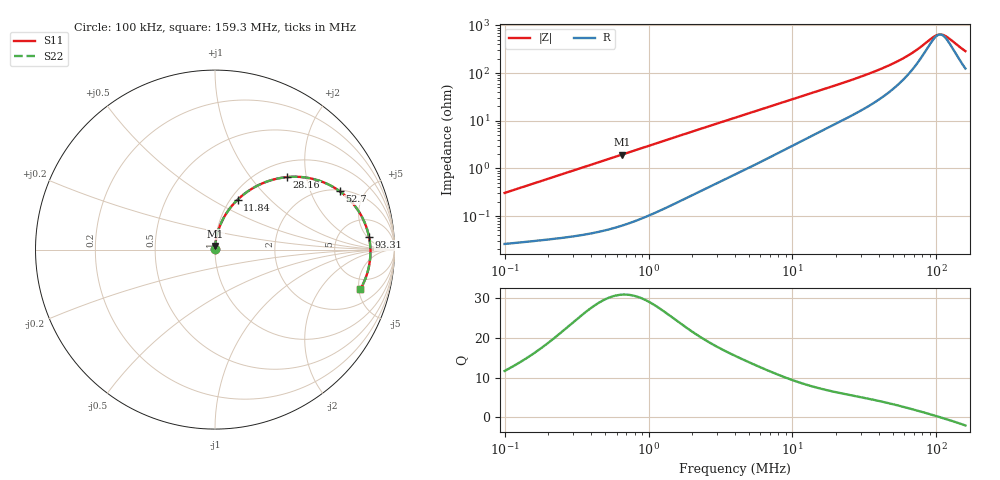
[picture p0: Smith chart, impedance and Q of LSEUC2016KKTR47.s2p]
! LSEUC2016KKTR47  S-PARAMETER MODEL  ( General Type )
! Model Generated by TAIYO YUDEN Corporation (http://www.ty-top.com)
! Version 1.0
! TAIYO YUDEN Control No. 220210
! Copyright(c) 2022 TAIYO YUDEN CO.,LTD. All Rights Reserved.
! Product Description (link to TY-COMPAS)
! https://ds.yuden.co.jp/TYCOMPAS/or/detail?pn=LSEUC2016KKTR47M&u=M
! Products Name : Inductors
! Characteristics :
!  Inductance : 0.47 uH , SRF(min) : -Hz , DC Resistance(max) : 0.026 Ohm
!  Rated Current : Saturation :6300 mA , Temp Rise : 4700 mA (40 degC)
!  Case Size : 2.0 x 1.6 / 0.079 x 0.063 [mm/inch] , Thickness : 1 / 0.039 [mm/inch]
!  (Conditions: Temperature = 25 degC , DC Bias Current/Voltage = 0A / 0V)
! External Node Assignments :
!  1  o---GGG---o  2
! GND o---------o GND
! Frequency Range : 0.1MHz  -  159.254811MHz  [ 402 STEP ]
# MHz S RI R 50
! Freq[MHz].  S11 Real  S11 Imag  S21 Real  S21 Imag  S12 Real  S12 Imag  S22 Real  S22 Imag
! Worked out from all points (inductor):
!   401 points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, 100 kHz to 159.3 MHz, reference 50 ohm
!   read as one part in series: L = 484 nH near 103.8 kHz
!   highest Q = 31 at 655.4 kHz (marker M1), where L = 476 nH
!   self-resonance near 106 MHz
!   S11 on the Smith chart (normalised r, x): 100 kHz: 1.00, +0.01; 11.84 MHz: 1.08, +0.66; 28.16 MHz: 1.30, +1.55; 52.7 MHz: 2.06, +3.26; 93.31 MHz: 10, +6; 159.3 MHz: 3.50, -5.21
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0.1  0.000271 0.00305  0.9997 -0.00305  0.9997 -0.00305  0.000271 0.00305
0.343835  0.000507 0.0103  0.9995 -0.0103  0.9995 -0.0103  0.000507 0.0103
0.655441  0.00102 0.0196  0.999 -0.0196  0.999 -0.0196  0.00102 0.0196
1.182227  0.00251 0.0351  0.9975 -0.0351  0.9975 -0.0351  0.00251 0.0351
2.295564  0.00782 0.0668  0.9922 -0.0668  0.9922 -0.0668  0.00782 0.0668
4.064915  0.021 0.1145  0.979 -0.1145  0.979 -0.1145  0.021 0.1145
7.33194  0.0578 0.1931  0.9422 -0.1931  0.9422 -0.1931  0.0578 0.1931
11.84009  0.1262 0.2783  0.8738 -0.2783  0.8738 -0.2783  0.1262 0.2783
13.72135  0.1579 0.306  0.8421 -0.306  0.8421 -0.306  0.1579 0.306
19.47584  0.2577 0.3664  0.7423 -0.3664  0.7423 -0.3664  0.2577 0.3664
28.15793  0.4019 0.4041  0.5981 -0.4041  0.5981 -0.4041  0.4019 0.4041
36.44803  0.5216 0.3989  0.4784 -0.3989  0.4784 -0.3989  0.5216 0.3989
47.17884  0.6444 0.3566  0.3556 -0.3566  0.3556 -0.3566  0.6444 0.3566
52.69613  0.6938 0.3259  0.3062 -0.3259  0.3062 -0.3259  0.6938 0.3259
61.06896  0.7532 0.2739  0.2468 -0.2739  0.2468 -0.2739  0.7532 0.2739
69.47957  0.7968 0.2191  0.2032 -0.2191  0.2032 -0.2191  0.7968 0.2191
93.31272  0.8582 0.0701  0.1418 -0.0701  0.1418 -0.0701  0.8582 0.0701
102.3215  0.865 0.0194  0.135 -0.0194  0.135 -0.0194  0.865 0.0194
112.2001  0.8656 -0.0319  0.1344 0.0319  0.1344 0.0319  0.8656 -0.0319
120.7853  0.8614 -0.073  0.1386 0.073  0.1386 0.073  0.8614 -0.073
147.9352  0.8293 -0.1826  0.1707 0.1826  0.1707 0.1826  0.8293 -0.1826
159.2548  0.8103 -0.22  0.1897 0.22  0.1897 0.22  0.8103 -0.22
